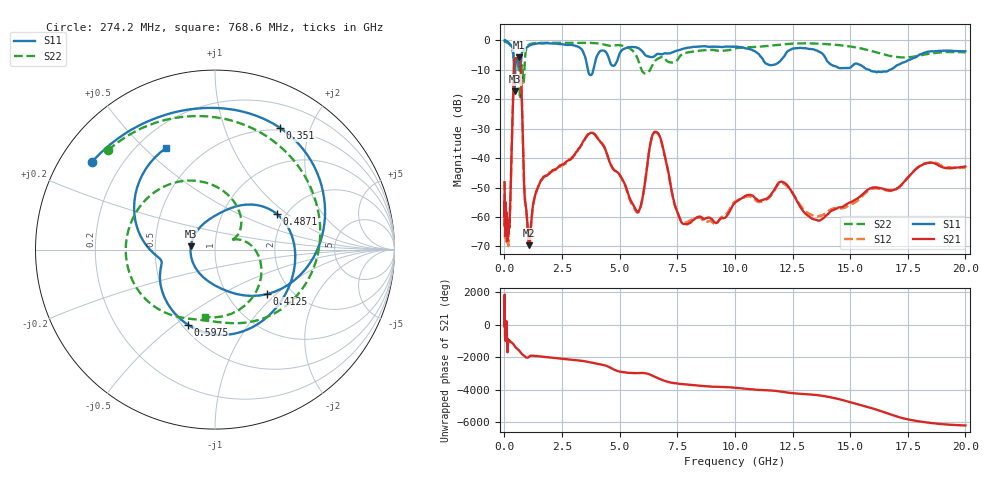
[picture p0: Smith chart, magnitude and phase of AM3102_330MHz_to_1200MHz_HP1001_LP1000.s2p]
! Date/Time: Tue, Sep 11, 2018 5:18 PM
! Network Analyzer: Agilent Technologies E8362B Rev: A.07.50.63
! Sweep from 0.010 to 20.000 GHz, 1601 Points, Sweep Type: LOG
! Power Supply: 4.949 V, 0.001 A
# Hz S DB R 50
!freq MagS11 AngS11 MagS21 AngS21 MagS12 AngS12 MagS22 AngS22
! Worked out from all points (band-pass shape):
!   1601 points, 10 MHz to 20 GHz, reference 50 ohm
!   highest |S21| = -5.66 dB at 617.7 MHz (marker M1); lowest = -69.7 dB at 1.077 GHz (marker M2)
!   |S21| within 3 dB of the highest: 421 MHz to 700 MHz (279 MHz wide, 49.8 % of centre)
!   lowest |S11| = -17.3 dB at 443 MHz (marker M3), VSWR 1.32, Z = 38.1 + j1.5 ohm
!   |S11| at or under -10 dB: 417.4 MHz to 472.5 MHz (55.09 MHz wide, 12.4 % of centre); 3.626 GHz to 3.859 GHz (233.8 MHz wide, 6.25 % of centre); 15.83 GHz to 16.72 GHz (883.4 MHz wide, 5.43 % of centre)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
!   |S22| runs from -19.9 to -0.2 dB; largest |S21 - S12| = 0.0099
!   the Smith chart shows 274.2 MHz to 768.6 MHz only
!   S11 on the Smith chart (normalised r, x): 274.2 MHz: 0.09, +0.32; 351 MHz: 0.47, +1.56; 412.5 MHz: 1.51, -0.88; 487.1 MHz: 1.79, +0.85; 597.5 MHz: 0.53, -0.56; 768.6 MHz: 0.31, +0.59
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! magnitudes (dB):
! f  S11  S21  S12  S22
! 10 MHz  0.0  -48.2  -47.8  -0.2
! 35.55 MHz  0.0  -62.8  -64.9  -0.4
! 126.4 MHz  -0.4  -66.0  -63.5  -0.8
! 167.3 MHz  -0.6  -64.7  -68.8  -1.0
! 274.2 MHz  -1.5  -50.3  -50.2  -1.8
! 351 MHz  -2.3  -26.6  -26.7  -3.4
! 412.5 MHz  -8.4  -10.0  -10.1  -6.5
! 443 MHz  -17.3  -6.6  -6.6  -8.0
! 447.2 MHz  -17.1  -6.4  -6.4  -8.0
! 487.1 MHz  -8.0  -6.0  -6.1  -6.5
! 597.5 MHz  -7.0  -5.7  -5.9  -8.2
! 617.7 MHz  -8.0  -5.7  -5.8  -10.0
! 768.6 MHz  -4.0  -23.1  -23.2  -8.4
! 869.7 MHz  -3.0  -51.6  -51.7  -10.1
! 1.077 GHz  -1.7  -69.7  -69.3  -1.4
! 1.59 GHz  -1.0  -47.6  -47.6  -0.8
! 3.811 GHz  -11.3  -31.4  -31.3  -0.9
! 5.652 GHz  -2.3  -56.8  -57.3  -4.3
! 6.58 GHz  -4.8  -31.1  -31.2  -6.6
! 7.882 GHz  -2.6  -62.4  -61.9  -4.2
! 13.68 GHz  -3.9  -61.2  -59.6  -1.1
! 20 GHz  -3.6  -42.8  -43.3  -4.0
